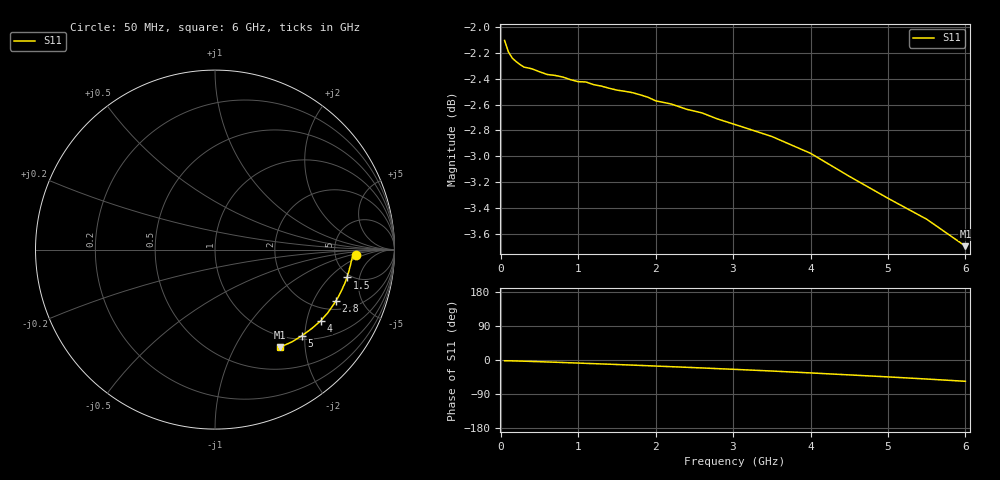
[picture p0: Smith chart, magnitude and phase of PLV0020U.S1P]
! Infineon Technologies  Discrete & RF Semiconductors
! BAR 64-04W /-05W /-06W
! Si PIN Diode in SOT323
! IF = 0.02 mA
! S-Parameters:  October  2008
# GHz  S  MA  R  50
!  f  S11
! GHz  MAG  ANG
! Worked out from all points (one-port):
!   34 points, 50 MHz to 6 GHz, reference 50 ohm
!   lowest |S11| = -3.7 dB at 6 GHz (marker M1), VSWR 4.77, Z = 40.9 - j77.6 ohm
!   |S11| at or under -10 dB: nowhere
!   S11 on the Smith chart (normalised r, x): 50 MHz: 8.13, -1.16; 1.5 GHz: 4.62, -3.28; 2.8 GHz: 2.49, -3.05; 4 GHz: 1.51, -2.42; 5 GHz: 1.08, -1.94; 6 GHz: 0.82, -1.55
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0.05  0.7848 -2.0
0.1  0.7768 -2.1
0.15  0.7726 -2.3
0.25  0.7681 -2.9
0.3  0.7664 -3.1
0.4  0.7653 -3.8
0.6  0.7614 -5.2
0.8  0.7597 -6.6
0.9  0.7579 -7.4
1  0.7566 -8.1
1.1  0.7563 -8.9
1.2  0.7546 -9.6
1.3  0.7536 -10.4
1.5  0.7509 -11.9
1.6  0.7501 -12.7
1.9  0.7462 -15.1
2  0.7438 -16.0
2.2  0.7417 -17.6
2.4  0.7382 -19.3
2.6  0.7358 -21.0
2.8  0.7319 -22.8
3  0.7287 -24.5
3.5  0.7206 -29.1
4  0.7099 -34.1
4.5  0.6955 -39.3
5  0.682 -44.6
5.5  0.6694 -50.2
6  0.6536 -56.2
